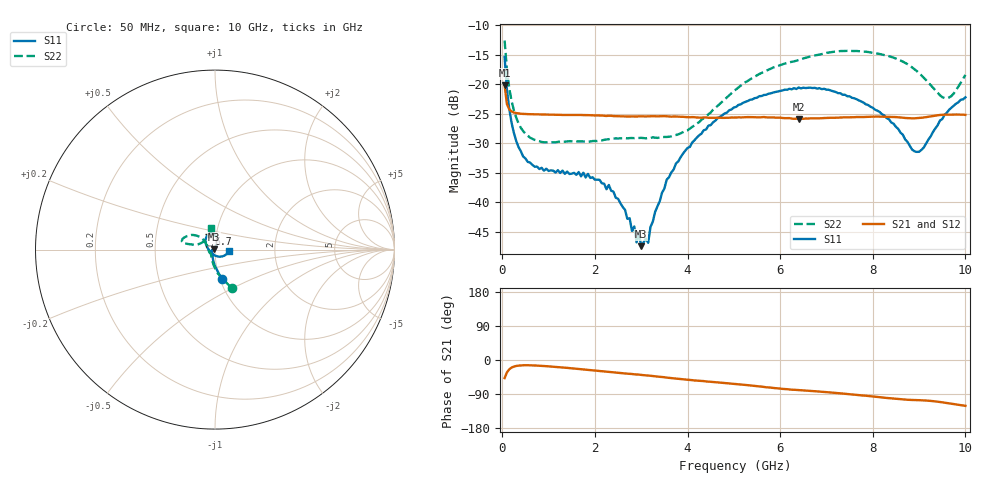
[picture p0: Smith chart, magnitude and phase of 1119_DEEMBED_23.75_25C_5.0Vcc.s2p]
!Hittite Microwave Corp.
!Digital Attenuator/PhaseShifter Rev 1.4.0
!Filename: C:\DATA\DATA\1119_DEEMBED_23.75_25C_5.0Vcc.s2p
!VNA ID: Agilent Technologies,N5224A,MY51441122,A.10.45.03
!Device type:
!2 Port Calibration.
!Temp(C): 25
!Lot Number:
!Serial Number:
!Operator:
!Misc:
!Attenuator:  23.750
# GHZ S DB R 50.0
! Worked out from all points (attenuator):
!   200 points, 50 MHz to 10 GHz, reference 50 ohm
!   highest |S21| = -20.17 dB at 50 MHz (marker M1); lowest = -25.9 dB at 6.4 GHz (marker M2)
!   lowest |S11| = -47.4 dB at 3 GHz (marker M3), VSWR 1.01, Z = 49.6 + j0.224 ohm
!   |S11| at or under -10 dB: start of sweep to end of sweep
!   |S22| runs from -29.8 to -12.6 dB; largest |S21 - S12| = 0.00019
!   S11 on the Smith chart (normalised r, x): 50 MHz: 1.02, -0.35; 6.7 GHz: 0.92, +0.16; 10 GHz: 1.17, -0.02
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0.05  -15.40 -77.0  -20.17 -47.6  -20.17 -47.7  -12.60 -66.8
0.1  -20.95 -90.8  -23.37 -32.8  -23.36 -32.7  -17.55 -83.5
0.2  -26.50 -105.7  -24.61 -20.1  -24.61 -20.0  -22.82 -100.2
0.45  -32.22 -129.2  -25.02 -13.9  -25.02 -14.0  -27.92 -120.9
0.9  -34.63 -153.2  -25.12 -15.9  -25.13 -15.9  -29.82 -135.2
1.75  -34.97 -164.2  -25.22 -24.9  -25.22 -25.0  -29.68 -139.9
2.3  -37.04 -171.9  -25.33 -31.5  -25.34 -31.6  -29.29 -148.2
2.8  -44.82 -178.7  -25.44 -36.9  -25.45 -37.1  -29.10 -155.3
2.85  -44.04 177.0  -25.45 -37.8  -25.46 -37.8  -29.12 -156.6
2.9  -46.75 168.3  -25.47 -38.1  -25.48 -38.1  -29.07 -157.9
2.95  -45.22 173.5  -25.43 -38.6  -25.44 -38.6  -29.09 -159.0
3  -47.39 148.2  -25.43 -39.4  -25.43 -39.4  -29.07 -160.5
3.15  -46.82 119.9  -25.43 -40.9  -25.44 -41.0  -29.08 -164.9
3.4  -39.80 90.8  -25.42 -44.2  -25.43 -44.3  -29.02 -172.3
3.95  -31.25 73.4  -25.55 -51.6  -25.55 -51.7  -27.90 165.5
5.05  -23.83 81.3  -25.63 -63.4  -25.65 -63.4  -20.86 139.4
6.4  -20.56 105.3  -25.86 -79.3  -25.88 -79.3  -15.91 150.5
6.7  -20.65 111.6  -25.77 -81.8  -25.78 -81.8  -15.21 154.4
8.35  -25.92 157.5  -25.52 -100.7  -25.53 -100.7  -15.26 168.2
8.999999  -31.42 -124.9  -25.71 -106.0  -25.71 -106.0  -18.13 167.4
9.6  -24.81 -39.5  -25.15 -113.6  -25.17 -113.6  -22.36 133.5
10  -22.22 -5.3  -25.19 -121.0  -25.19 -121.0  -18.43 99.7
